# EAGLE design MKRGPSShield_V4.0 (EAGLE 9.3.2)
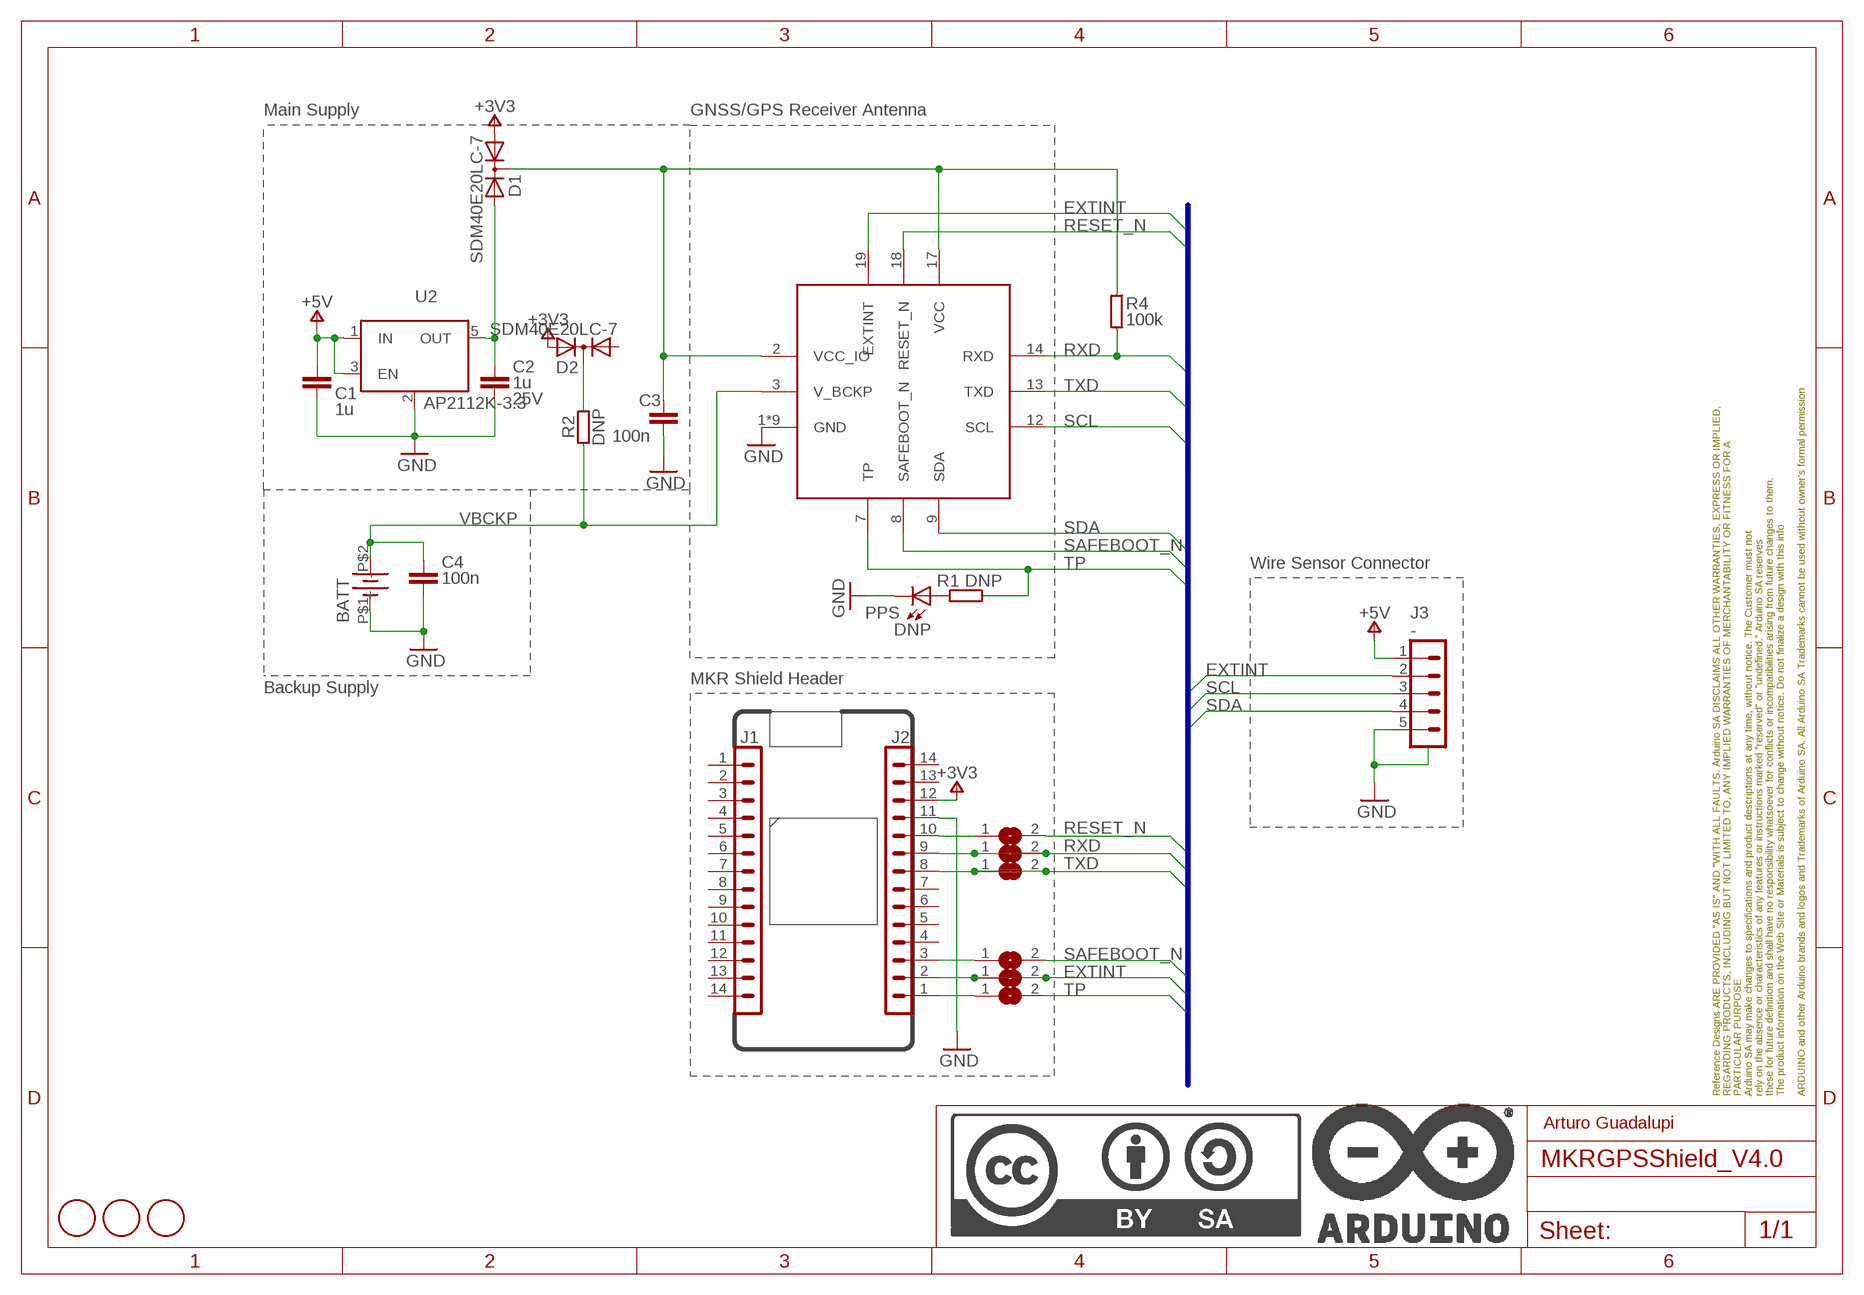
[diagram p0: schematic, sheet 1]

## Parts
BATT  BATT-HOLDER_12MM  [BATT-HOLDER_12MM]
C1  1u  C-1UF-0402  [0402-1005X55N]
C2  1u  C-1UF-0402  [0402-1005X55N]
C3  100n  C-100NF-0402  [0402-1005X55N]
C4  100n  C-100NF-0402  [0402-1005X55N]
D1  SDM40E20LC-7  A2K_SOT-323  [SOT65P210X110-3N]
D2  SDM40E20LC-7  A2K_SOT-323  [SOT65P210X110-3N]
FD1  DNP  FIDUCIAL-1.5MM  [FD-1-1.5]
FD2  DNP  FIDUCIAL-1.5MM  [FD-1-1.5]
FD3  DNP  FIDUCIAL-1.5MM  [FD-1-1.5]
FRAME1  DNP  A4L-LOC  [FRAME]
IC1  SAM-M8Q  [UBLOXLIB_SAM-M8Q]
J1  -  PINHD-1X14-SM-MALE/FEMALE-6_5VTH-SMD  [1X14_SMD_TH]
J2  -  PINHD-1X14-SM-MALE/FEMALE-AREF_5TH-SMD  [1X14_SMD_TH]
J3  -  SM05B-SRSS-TB  [SM05B-SRSS-TB]
PPS  DNP  LED-DNP-0603  [LEDC1608X80N-AK]
R1  DNP  R-DNP-0402  [0402-1005X55N]
R2  DNP  R-DNP-0402  [0402-1005X55N]
R4  100k  R-100K-0402  [0402-1005X55N]
SJ1  DNP  SJ  [SJ]
SJ2  DNP  SJ  [SJ]
SJ5  DNP  SJ  [SJ]
SJ6  DNP  SJ  [SJ]
SJ7  DNP  SJ  [SJ]
SJ8  DNP  SJ  [SJ]
U2  AP2112K-3.3  [SOT25]

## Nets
+3V3: D1.1(A1) D2.2(A2) J2.12
+5V: C1.1 J3.1 U2.1(IN) U2.3(EN)
EXTINT: IC1.19(EXTINT) J2.2 J3.2 SJ1.1 SJ1.2
GND: BATT.P$1(-) C1.2 C2.2 C3.2 C4.2 IC1.1(GND) IC1.4(GND) IC1.5(GND) IC1.6(GND) IC1.10(GND) IC1.11(GND) IC1.15(GND) IC1.16(GND) IC1.20(GND) J2.11 J3.5 J3.SH1(SH) J3.SH2(SH) PPS.C U2.2(GND/ADJ)
N$1: J2.1 SJ2.1
N$2: D2.3(K) R2.2
N$3: J2.10 SJ7.1
N$4: J2.3 SJ8.1
N$7: PPS.A R1.2
N$10: C2.1 D1.2(A2) U2.5(OUT)
RESET_N: IC1.18(RESET_N) SJ7.2
RXD: IC1.14(RXD) J2.9 R4.1 SJ6.1 SJ6.2
SAFEBOOT_N: IC1.8(SAFEBOOT_N) SJ8.2
SCL: IC1.12(SCL) J3.3
SDA: IC1.9(SDA) J3.4
TP: IC1.7(TP) R1.1 SJ2.2
TXD: IC1.13(TXD) J2.8 SJ5.1 SJ5.2
VBCKP: BATT.P$2(+) C4.1 IC1.3(V_BCKP) R2.1
VCC: C3.1 D1.3(K) IC1.2(VCC_IO) IC1.17(VCC) R4.2
Unconnected: D2.1(A1) J1.1 J1.2 J1.3 J1.4 J1.5 J1.6 J1.7 J1.8 J1.9 J1.10 J1.11 J1.12 J1.13 J1.14 J2.4 J2.5 J2.6 J2.7 J2.13 J2.14

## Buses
+3V3,+5V,EXTINT,GND,N$1,N$3,N$4,N$5,N$7,N$8,N$10,RESET_N,RXD,SAFEBOOT_N,SCL,SDA,TP,TXD,VBCKP,VCC

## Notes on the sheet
- Main Supply | GNSS/GPS Receiver Antenna
- Wire Sensor Connector
- MKR Shield Header
- Backup Supply
- Arturo Guadalupi

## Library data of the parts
BATT = Arduino-connectors:BATT-HOLDER_12MM: 12.5mm coincell battery holder; CODE-ARDUINO: A5379; DATASHEET: http://keyelco.com/userAssets/file/M65p2.pdf; DISTRIBUTOR-LINK: https://www.digikey.it/product-detail/it/keystone-electronics/1056TR/36-1056CT-ND/4772075; DISTRIBUTOR-PN: 36-1056CT-ND; MANUFACTURER: Keystone; MANUFACTURER-PN: 1056TR
C1 C2 = Arduino-rcl:C: SMD Capacitor; CODE-ARDUINO: 0133; DATASHEET: http://search.murata.co.jp/Ceramy/image/img/A01X/partnumbering_e_01.pdf; DISTRIBUTOR-LINK: http://www.digikey.com/product-detail/en/murata-electronics-north-america/GRM155R61E105KA12D/490-10017-1-ND/5026367; DISTRIBUTOR-PN: 490-10017-1-ND; MANUFACTURER: Murata; MANUFACTURER-PN: GRM155R61E105KA12D; NOTE: -; VOLTAGE: 25V
C3 = Arduino-rcl:C: SMD Capacitor; CODE-ARDUINO: 0132; DATASHEET: http://www.tdk.com/pdf/TDKMLCCCapRange.pdf; DISTRIBUTOR-LINK: http://www.digikey.com/product-detail/en/tdk-corporation/C1005X5R1H104K050BB/445-5942-1-ND/2443982; DISTRIBUTOR-PN: 445-5942-1-ND; MANUFACTURER: TDK; MANUFACTURER-PN: C1005X5R1H104K050BB; NOTE: -
C4 = Arduino-rcl:C: SMD Capacitor; CODE-ARDUINO: 0132; DATASHEET: http://www.tdk.com/pdf/TDKMLCCCapRange.pdf; DISTRIBUTOR-LINK: http://www.digikey.com/product-detail/en/tdk-corporation/C1005X5R1H104K050BB/445-5942-1-ND/2443982; DISTRIBUTOR-PN: 445-5942-1-ND; MANUFACTURER: TDK; MANUFACTURER-PN: C1005X5R1H104K050BB; NOTE: -; VOLTAGE: 25V
D1 D2 = Arduino-diodes:A2K_; CODE-ARDUINO: A5457; DATASHEET: https://www.diodes.com/assets/Datasheets/ds30298.pdf; DISTRIBUTOR-LINK: https://www.digikey.com/product-detail/en/diodes-incorporated/SDM40E20LC-7/SDM40E20LC-7DICT-ND/2260642; DISTRIBUTOR-PN: SDM40E20LC-7DICT-ND; MANUFACTURER: Diodes Incorporated; MANUFACTURER-PN: SDM40E20LC-7; NOTE: NO
FD1-FD3 = Arduino-utility:FIDUCIAL: Fiducial mount; CODE-ARDUINO: DNP; DATASHEET: DNP; DISTRIBUTOR-LINK: DNP; DISTRIBUTOR-PN: DNP; MANUFACTURER: DNP; MANUFACTURER-PN: DNP
FRAME1 = Arduino-utility:A4L-LOC; CODE-ARDUINO: DNP; DATASHEET: DNP; DISTRIBUTOR-LINK: DNP; DISTRIBUTOR-PN: DNP; MANUFACTURER: DNP; MANUFACTURER-PN: DNP; NOTE: DNP
IC1 = Arduino-ucs&SoCs:SAM-M8Q: u-blox SAM GNSS antenna module; CODE-ARDUINO: SAM-M8Q-0-10; DATASHEET: https://www.u-blox.com/sites/default/files/SAM-M8Q_DataSheet_%28UBX-16012619%29.pdf; DISTRIBUTOR-LINK: https://www.digikey.com/product-detail/en/u-blox-america-inc/SAM-M8Q-0-10/672-1054-1-ND/7393573; DISTRIBUTOR-PN: 672-1054-1-ND; MANUFACTURER: U-Blox; MANUFACTURER-PN: SAM-M8Q-0-10; NOTE: NO
J1 = Arduino-connectors:PINHD-1X14-SM: PIN HEADER; CODE-ARDUINO: A5272; DATASHEET: -; DISTRIBUTOR-LINK: -; DISTRIBUTOR-PN: -; MANUFACTURER: -; MANUFACTURER-PN: -
J2 = Arduino-connectors:PINHD-1X14-SM: PIN HEADER; CODE-ARDUINO: A5273; DATASHEET: -; DISTRIBUTOR-LINK: -; DISTRIBUTOR-PN: -; MANUFACTURER: -; MANUFACTURER-PN: -
J3 = Arduino-connectors:SM05B-SRSS-TB: CONN HEADER SH 5POS SIDE 1MM TIN Datasheet; CODE-ARDUINO: 2353; DATASHEET: http://www.jst-mfg.com/product/pdf/eng/eSH.pdf; DISTRIBUTOR-LINK: http://www.digikey.com/product-detail/en/jst-sales-america-inc/SM05B-SRSS-TB(LF)(SN)/455-1805-1-ND/926876; DISTRIBUTOR-PN: 455-1805-1-ND; MANUFACTURER: JST; MANUFACTURER-PN: SM05B-SRSS-TB
PPS = Arduino-diodes:LED: LED; CODE-ARDUINO: DNP; DATASHEET: DNP; DISTRIBUTOR-LINK: DNP; DISTRIBUTOR-PN: DNP; MANUFACTURER: DNP; MANUFACTURER-PN: DNP
R1 = Arduino-rcl:R: SMD Resistor; CODE-ARDUINO: DNP; DATASHEET: DNP; DISTRIBUTOR-LINK: DNP; DISTRIBUTOR-PN: DNP; MANUFACTURER: DNP; MANUFACTURER-PN: DNP; _RESTRICTIONS: NO
R2 = Arduino-rcl:R: SMD Resistor; CODE-ARDUINO: DNP; DATASHEET: DNP; DISTRIBUTOR-LINK: DNP; DISTRIBUTOR-PN: DNP; MANUFACTURER: DNP; MANUFACTURER-PN: DNP; NOTE: NO
R4 = Arduino-rcl:R: SMD Resistor; CODE-ARDUINO: 0134; DATASHEET: www.yageo.com.tw/exep/pages/download/literatures/PYu-R_INT-thick_7.pdf; DISTRIBUTOR-LINK: http://www.digikey.com/product-detail/en/yageo/RC0402FR-07100KL/311-100KLRCT-ND/729473; DISTRIBUTOR-PN: 311-100KLRCT-ND; MANUFACTURER: Yageo; MANUFACTURER-PN: RC0402FR-07100KL; MPN: RC0402FR-07100KL; NOTE: NO
SJ1 SJ2 SJ5-SJ8 = Arduino-utility:SJ: SMD solder JUMPER; CODE-ARDUINO: DNP; DATASHEET: DNP; DISTRIBUTOR-LINK: DNP; DISTRIBUTOR-PN: DNP; MANUFACTURER: DNP; MANUFACTURER-PN: DNP
U2 = Arduino-ICs:AP2112K-3.3: IC REG LINEAR 3.3V 600mA SOT25; CODE-ARDUINO: 2199; DATASHEET: https://www.diodes.com/assets/Datasheets/AP2112.pdf; DISTRIBUTOR-LINK: https://www.digikey.com/product-detail/en/diodes-incorporated/AP2112K-3.3TRG1/AP2112K-3.3TRG1DITR-ND/4470746; DISTRIBUTOR-PN: AP2112K-3.3TRG1DITR-ND; MANUFACTURER: Diodes Inc; MANUFACTURER-PN: AP2112K-3.3TRG1; NOTE: NO

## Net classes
0 default: width 0.25 mm, drill 0.25 mm

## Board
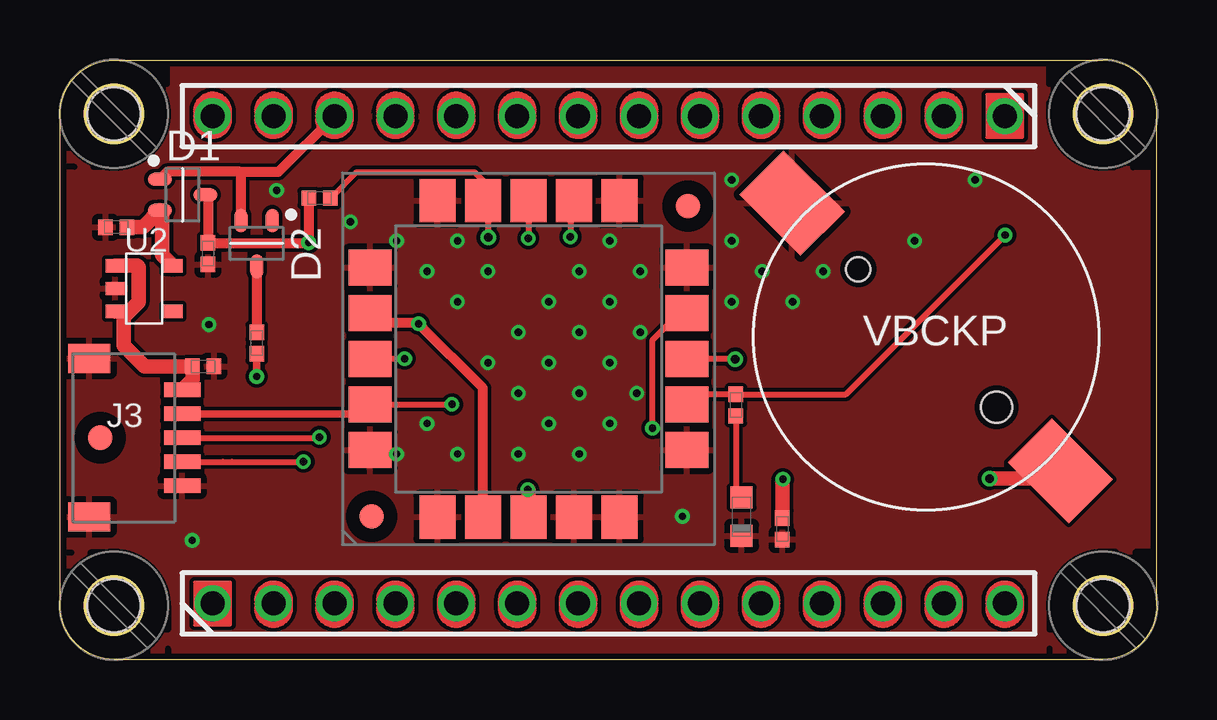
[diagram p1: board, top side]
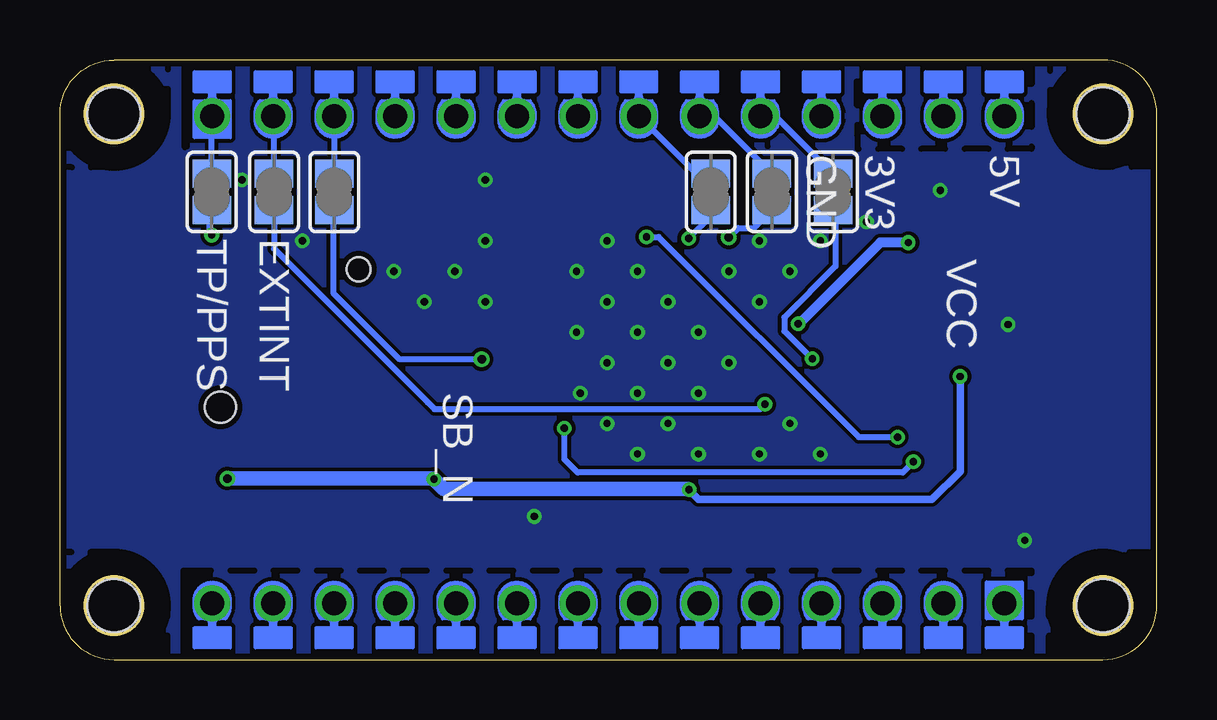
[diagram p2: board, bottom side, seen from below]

Size 45.73 x 25 mm. Coordinates in mm from the lower left corner, seen from the top.
Outline: 43.48,0 2.25,0 arc-90 0,2.25 0,22.75 arc-90 2.25,25 43.48,25 arc-90 45.73,22.75 45.73,2.25 arc-90 43.48,0
Copper layers (1*16): Top 0.035mm / dielectric 1.5mm / Bottom 0.035mm
Design rules "SeeedStudio_2layers": minimum track width 6mil, minimum drill 12mil, track to track 6mil, track to pad 6mil, pad to pad 6mil, via to via 6mil, smd to smd 0mil, copper to edge 10mil, drill to drill 10mil, minimum pad ring 10mil, minimum via ring 6mil, stop-mask expansion 2mil, vias tented up to drill 100mil, thermal gap 10mil
Holes 2.2 mm at 2.25,2.25 43.48,2.25 43.48,22.75 2.25,22.75
tRestrict: area 0,0 to 4.5,4.5; area 0,20.5 to 4.5,25; area 41.2,20.5 to 45.7,25; area 41.2,0 to 45.7,4.5; 17 lines
bRestrict: area 0,0 to 4.5,4.5; area 41.2,0 to 45.7,4.5; area 41.2,20.5 to 45.7,25; area 0,20.5 to 4.5,25; 104 lines

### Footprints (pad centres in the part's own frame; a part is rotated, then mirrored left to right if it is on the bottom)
BATT-HOLDER_12MM = smd 3.6 x 2.6: P$1 -7.9,0; P$2 7.9,0 | hole 1: -4,0 | hole 1.3: 4.15,0
0402-1005X55N = smd 0.62 x 0.62: 1 -0.45,0; 2 0.45,0
SOT65P210X110-3N = smd 1 x 0.55: 1 -0.95,0.65; 2 -0.95,-0.65; 3 0.95,0
FD-1-1.5 = smd 1.016 x 1.016: P$1 0,0
UBLOXLIB_SAM-M8Q = smd 1.8 x 1.5: 1 -6.6,3.8; 2 -6.6,1.9; 3 -6.6,0; 4 -6.6,-1.9; 5 -6.6,-3.8; 11 6.6,-3.8; 12 6.6,-1.9; 13 6.6,0; 14 6.6,1.9; 15 6.6,3.8 | smd 1.5 x 1.8: 6 -3.8,-6.6; 7 -1.9,-6.6; 8 0,-6.6; 9 1.9,-6.6; 10 3.8,-6.6; 16 3.8,6.6; 17 1.9,6.6; 18 0,6.6; 19 -1.9,6.6; 20 -3.8,6.6
1X14_SMD_TH = drill 1: 1 0,0; 2 2.54,0; 3 5.08,0; 4 7.62,0; 5 10.16,0; 6 12.7,0; 7 15.24,0; 8 17.78,0; 9 20.32,0; 10 22.86,0; 11 25.4,0; 12 27.94,0; 13 30.48,0; 14 33.02,0
SM05B-SRSS-TB = smd 0.6 x 1.55: 1 -2,2.425; 2 -1,2.425; 3 0,2.425; 4 1,2.425; 5 2,2.425 | smd 1.2 x 1.8: SH1 -3.3,-1.45; SH2 3.3,-1.45
LEDC1608X80N-AK = smd 0.9 x 0.95: A 0.8,0; C -0.8,0
SJ = smd 1.168 x 1.6: 1 -0.762,0; 2 0.762,0
SOT25 = smd 0.55 x 0.8: 1 0.95,1.2; 2 0,1.2; 3 -0.95,1.2; 4 -0.95,-1.2; 5 0.95,-1.2

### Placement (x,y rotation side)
BATT  36.11,13.45 315 top
C1  5.97,12.22 0 top
C2  2.35,18.02 180 top
C3  6.17,16.93 270 top
C4  30.11,5.45 270 top
D1  5.11,19.38 0 top
D2  8.2,17.35 270 top
FD1  12.98,5.96 90 top
FD2  26.18,18.9 90 top
FD3  1.68,9.25 0 top
FRAME1  0,0 0 top
IC1  19.53,12.54 90 top
J1  6.36,2.34 0 top
J2  39.38,22.66 180 top
J3  2.67,9.25 270 top
PPS  28.41,5.96 90 top
R1  28.17,10.61 270 top
R2  8.2,13.2 90 top
R4  10.82,19.24 180 top
SJ1  36.8,19.5 270 bottom
SJ2  39.4,19.5 270 bottom
SJ5  18.6,19.5 270 bottom
SJ6  16.05,19.5 270 bottom
SJ7  13.5,19.5 270 bottom
SJ8  34.29,19.49 270 bottom
U2  3.51,15.47 90 top
U$5  [MH_RND_F_2.2MM_NM]  2.25,2.25 90 top
U$6  [MH_RND_F_2.2MM_NM]  2.25,22.75 90 top
U$7  [MH_RND_F_2.2MM_NM]  43.48,22.75 90 top
U$8  [MH_RND_F_2.2MM_NM]  43.48,2.25 90 top

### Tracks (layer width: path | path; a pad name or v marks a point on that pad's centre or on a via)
+3V3
  Top 0.406: D2.2 7.55,20.28 7.5,20.33 | 7.5,20.33 4.46,20.33 D1.1 | 7.5,20.33 9.11,20.33 J2.12
+5V
  Top 0.61: 5,11.25 J3.1 5.53,11.68 C1.1 3.52,12.22 2.65,13.1 2.65,14.28 2.89,14.52 | 2.89,14.52 U2.3 | 2.89,14.52 3.27,14.9 3.27,16.37 3.23,16.42 U2.1
EXTINT  (via drill 0.3)
  Top 0.254: IC1.19 v16.34,10.64
  Top 0.305: J3.2 12.54,10.25 IC1.19
  Bottom 0.25: J2.2 36.8,22.62 SJ1.1 SJ1.2 36.8,17.13 30.39,10.71
  Bottom 0.254: v16.34,10.64 16.54,10.44 30.11,10.44 30.39,10.71
GND  (via drill 0.3)
  other vias: 28,20 28,17.46 28,14.92 29.27,16.19 30.54,14.92 31.81,16.19 35.62,17.46 38.14,20 16.57,14.92 15.3,16.19 17.84,16.19 16.57,17.46 20.38,14.92 22.92,14.92 21.65,13.65 20.38,12.38 22.92,12.38 21.65,11.11 19.11,13.65 24.19,13.65 19.11,11.11 24.04,11.11 19.11,8.57 21.65,8.57 20.38,9.84 22.92,9.84 16.57,8.57 15.3,9.84 21.65,16.19 24.19,16.19 17.84,12.38 14.03,8.57 14.03,17.46 12.11,18.25 9.03,19.56 25.95,5.97 5.51,4.97 6.21,13.97 22.92,17.46
  pour Bottom: 0,0 0,25 45.73,25 45.73,0
  pour Top: 0,-0.1 0,24.9 12.72,25 45.73,25 45.73,0
N$1
  Bottom 0.25: SJ2.1 39.4,22.64 J2.1
N$2
  Top 0.406: D2.3 R2.2
N$3
  Bottom 0.25: SJ7.1 15.9,22.66 J2.10
N$4
  Bottom 0.25: J2.3 SJ8.1
N$7
  Top 0.254: R1.2 28.18,7 PPS.A
N$10
  Top 0.61: U2.5 4.25,16.87 4.25,18.64 D1.2 3.46,18.03 C2.1
RESET_N  (via drill 0.3)
  Top 0.254: v14.36,12.55 14.35,12.54 IC1.18
  Bottom 0.254: SJ7.2 13.4,18.64 13.4,16.4 15.53,14.27 15.53,13.7 14.39,12.55 v14.36,12.55
RXD  (via drill 0.35)
  Top 0.25: v17.85,17.6 17.85,18.92 IC1.14
  Top 0.254: IC1.14 17.63,19.97 17.29,20.32 12.34,20.32 11.33,19.31 11.3,19.31 11.3,19.26 R4.1
  Bottom 0.25: v17.85,17.6 17.45,18 16.79,18 SJ6.2 SJ6.1 18.45,22.66 J2.9
SAFEBOOT_N  (via drill 0.35)
  Top 0.25: IC1.8 28.13,12.54 v28.15,12.52
  Bottom 0.25: SJ8.2 34.33,18.69 34.33,15.29 31.56,12.52 v28.15,12.52
SCL  (via drill 0.3)
  Top 0.25: v10.81,9.28 10.79,9.25 J3.3
  Top 0.254: IC1.12 21.27,18.98 v21.27,17.62
  Bottom 0.254: v10.81,9.28 12.43,9.28 20.77,17.62 v21.27,17.62
SDA  (via drill 0.3)
  Top 0.25: 25.97,14.6 IC1.9 | J3.4 6.8,8.25 7.17,8.25
  Top 0.254: 6.8,8.25 v10.15,8.25 | 25.97,14.6 24.7,13.33 v24.7,9.65
  Bottom 0.254: v10.15,8.25 10.6,7.8 24.15,7.8 24.7,8.35 v24.7,9.65
TP  (via drill 0.3)
  Top 0.254: IC1.7 26.55,11.05 R1.1 32.76,11.05 v39.4,17.7
  Bottom 0.25: 39.49,18.65 SJ2.2
  Bottom 0.254: v39.4,17.7 39.49,17.79 39.49,18.65
TXD  (via drill 0.3)
  Top 0.254: 19.52,19.13 IC1.13 19.53,17.57 v19.52,17.56
  Bottom 0.25: 19.2,20.26 J2.8
  Bottom 0.254: v19.52,17.56 18.6,18.48 SJ5.2 SJ5.1 19.2,20.26
VBCKP  (via drill 0.3, 0.35)
  Top 0.25: BATT.P$2 42.01,7.55
  Top 0.305: v8.2,11.8 R2.1
  Top 0.61: IC1.3 19.53,7.08 v19.5,7.08 | 42.01,7.55 v38.75,7.55 v38.75,7.54 | v30.13,7.52 30.11,7.49 C4.1
  Bottom 0.305: v19.5,7.08 19.1,6.68 9.37,6.68 8.2,7.85 v8.2,11.8
  Bottom 0.61: v19.5,7.08 19.54,7.12 29.73,7.12 v30.13,7.52 30.17,7.55 38.65,7.55 38.66,7.54 v38.75,7.54
VCC  (via drill 0.3)
  Top 0.254: 13.33,14.03 IC1.17
  Top 0.406: 6.17,17.46 6.09,17.46 | 6.17,17.46 C3.1 10.35,17.38 10.35,17.37 v10.36,17.39 v10.37,17.39 R4.2 | D1.3 6.17,19.27 6.17,17.46 | IC1.2 17.63,11.32 v14.95,14 14.92,14.03 13.33,14.03
  Bottom 0.406: v10.36,17.39 11.53,17.39 14.92,14 v14.95,14

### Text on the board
tPlace: VBCKP
bPlace: 5V | 3V3 | GND | EXTINT | TP/PPS | VCC | SB_N
tDocu: IC1

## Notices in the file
MKRGPSShield_V4.0.brd:
Copyright (c) 2016-2017 Arduino LLC. All right reserved. EAGLE Design Rules
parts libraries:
Arduino-connectors: Copyright (c) 2016-2017 Arduino LLC. All right reserved.
